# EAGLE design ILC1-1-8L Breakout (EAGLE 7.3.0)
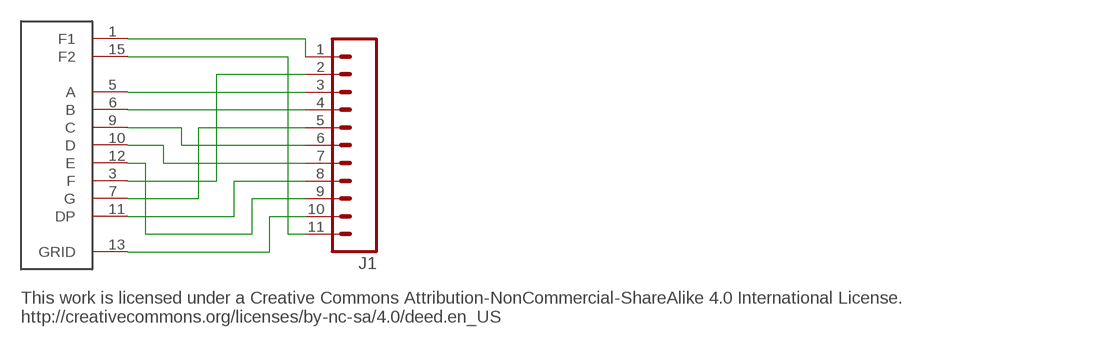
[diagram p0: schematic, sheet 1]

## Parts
J1  M11PTH  [1X11]
U$2  ILC1-1_8L  [ILC1-1_8L]

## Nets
N$1: J1.2 U$2.3(F)
N$2: J1.1 U$2.1(F1)
N$3: J1.3 U$2.5(A)
N$4: J1.4 U$2.6(B)
N$5: J1.5 U$2.7(G)
N$6: J1.6 U$2.9(C)
N$7: J1.7 U$2.10(D)
N$8: J1.8 U$2.11(DP)
N$9: J1.9 U$2.12(E)
N$10: J1.11 U$2.15(F2)
N$11: J1.10 U$2.13(GRID)

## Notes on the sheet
- This work is licensed under a Creative Commons Attribution-NonCommercial-ShareAlike 4.0 International License.
  http://creativecommons.org/licenses/by-nc-sa/4.0/deed.en_US

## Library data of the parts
J1 = SparkFun-Connectors:M11: Header 11 Standard 11-pin 0.1" header. Use with straight break away headers (SKU : PRT-00116), right angle break away headers (PRT-00553), swiss pins (PRT-00743), machine pins (PRT-00117), and female headers (PRT-00115).
U$2 = ILC1-1_8L:ILC1-1_8L

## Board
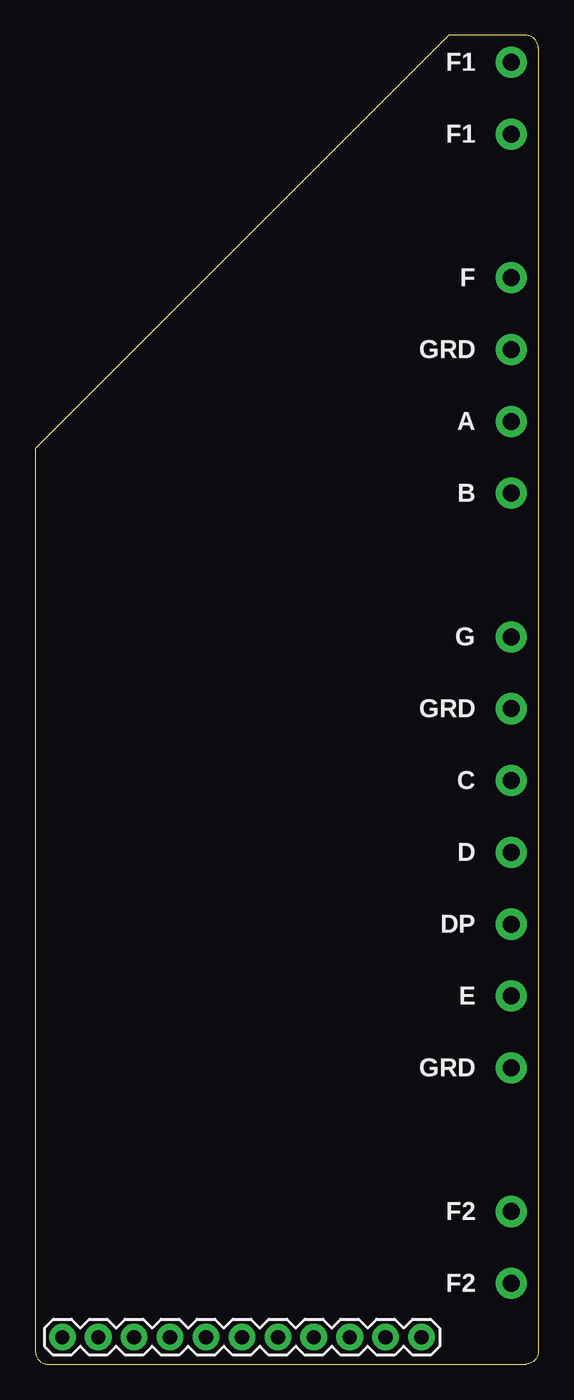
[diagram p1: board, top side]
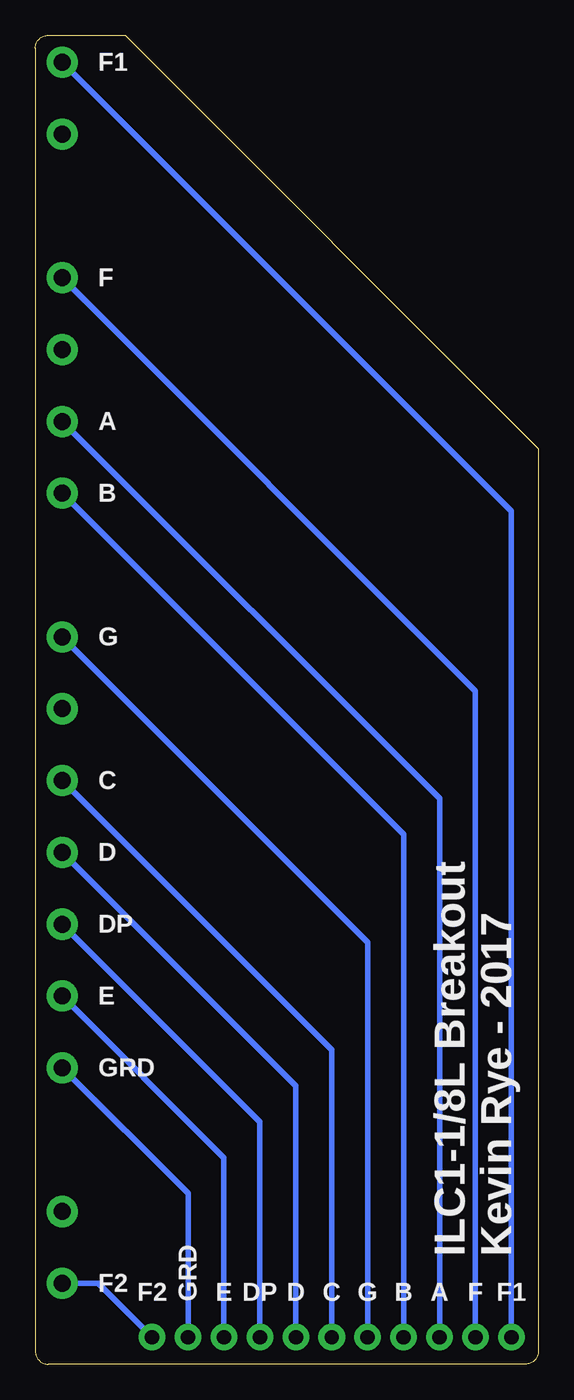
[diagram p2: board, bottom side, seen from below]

Size 35.56 x 93.98 mm. Coordinates in mm from the lower left corner, seen from the top.
Outline: 35.56,93.08 35.56,0.9 arc-90 34.66,0 0.9,0 arc-90 0,0.9 0,64.76 29.22,93.98 34.66,93.98 arc-90 35.56,93.08
Copper layers (1*16): Top 0.0356mm / dielectric 1.5011mm / Bottom 0.0356mm
Design rules "oshpark-2layer": minimum track width 6mil, minimum drill 13mil, track to track 6mil, track to pad 6mil, pad to pad 6mil, via to via 6mil, smd to smd 6mil, copper to edge 15mil, drill to drill 6mil, minimum pad ring 7mil, minimum via ring 7mil, stop-mask expansion 2.5mil, vias tented up to drill 0mil, thermal gap 10mil

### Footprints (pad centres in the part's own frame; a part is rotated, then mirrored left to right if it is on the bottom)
1X11 = drill 1.016 pad 1.88: 1 0,0; 2 2.54,0; 3 5.08,0; 4 7.62,0; 5 10.16,0; 6 12.7,0; 7 15.24,0; 8 17.78,0; 9 20.32,0; 10 22.86,0; 11 25.4,0
ILC1-1_8L = drill 1.2 pad 2.2: 1 0,86.36; 2 0,81.28; 3 0,71.12; 4 0,66.04; 5 0,60.96; 6 0,55.88; 7 0,45.72; 8 0,40.64; 9 0,35.56; 10 0,30.48; 11 0,25.4; 12 0,20.32; 13 0,15.24; 14 0,5.08; 15 0,0

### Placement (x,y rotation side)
J1  1.91,1.91 0 top
U$2  33.66,5.71 0 top

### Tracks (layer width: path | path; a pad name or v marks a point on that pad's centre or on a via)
N$1
  Bottom 0.406: J1.2 4.45,47.62 U$2.3
N$2
  Bottom 0.406: U$2.1 1.91,60.32 J1.1
N$3
  Bottom 0.406: J1.3 6.98,40 U$2.5
N$4
  Bottom 0.406: J1.4 9.53,37.46 U$2.6
N$5
  Bottom 0.406: J1.5 12.07,29.84 U$2.7
N$6
  Bottom 0.406: J1.6 14.61,22.22 U$2.9
N$7
  Bottom 0.406: J1.7 17.15,19.68 U$2.10
N$8
  Bottom 0.406: J1.8 19.69,17.14 U$2.11
N$9
  Bottom 0.406: J1.9 22.23,14.61 U$2.12
N$10
  Bottom 0.406: J1.11 31.12,5.71 U$2.15
N$11
  Bottom 0.406: J1.10 24.77,12.07 U$2.13

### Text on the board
Unrouted: This work is licensed under a Creative Commons Attribution-NonCommercial-ShareAlike 4.0 International License. / http://creativecommons.org/licenses/by-nc-sa/4.0/deed.en_US
bPlace: ILC1-1/8L Breakout / Kevin Rye - 2017
bNames: F1 | F | A | B | G | C | D | DP | E | GRD | F2 | F1 | F | A | B | G | C | D | DP | E | GRD | F2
